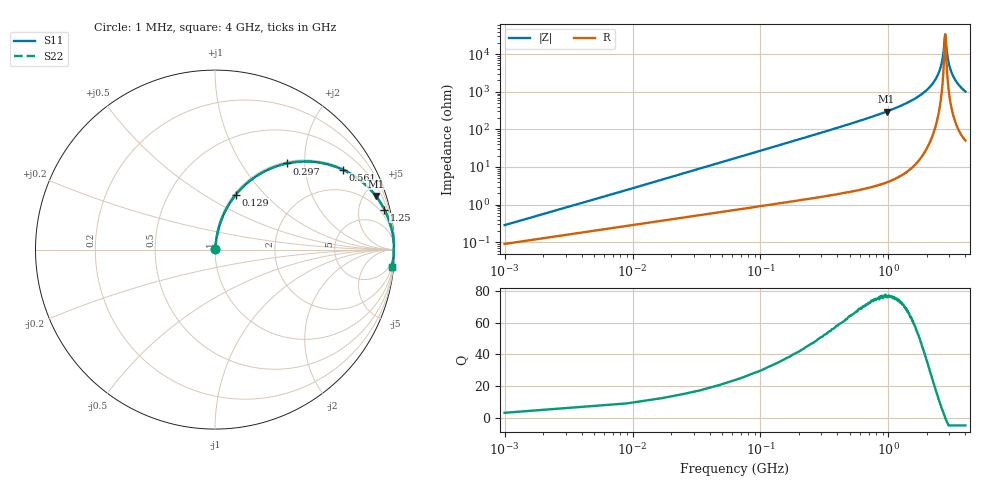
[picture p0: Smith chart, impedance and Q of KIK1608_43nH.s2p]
!version-2
!date-01.2022
!Series
# MHz S RI R 50
!Freq ReS11 ImS11 ReS21 ImS21 ReS12 ImS12 ReS22 ImS22
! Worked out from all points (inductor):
!   501 points, 1 MHz to 4 GHz, reference 50 ohm
!   read as one part in series: L = 43 nH near 17 MHz
!   highest Q = 76.7 at 969 MHz (marker M1), where L = 48.9 nH
!   self-resonance near 2.775 GHz
!   S11 on the Smith chart (normalised r, x): 1 MHz: 1.00, +0.01; 129 MHz: 1.02, +0.70; 297 MHz: 1.03, +1.62; 561 MHz: 1.05, +3.16; 1.25 GHz: 1.12, +8.45; 4 GHz: 2, -20
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1  0.000914 0.0027  0.9991 -0.0027  0.9991 -0.0027  0.000914 0.0027
25  0.009 0.0666  0.991 -0.0666  0.991 -0.0666  0.009 0.0666
41  0.0177 0.1082  0.9823 -0.1082  0.9823 -0.1082  0.0177 0.1082
73  0.0444 0.1872  0.9556 -0.1872  0.9556 -0.1872  0.0444 0.1872
129  0.1159 0.3056  0.8841 -0.3056  0.8841 -0.3056  0.1159 0.3056
297  0.3992 0.48  0.6008 -0.48  0.6008 -0.48  0.3992 0.48
561  0.7112 0.4458  0.2888 -0.4458  0.2888 -0.4458  0.7112 0.4458
673  0.7853 0.4037  0.2147 -0.4037  0.2147 -0.4037  0.7853 0.4037
969  0.8956 0.2993  0.1044 -0.2993  0.1044 -0.2993  0.8956 0.2993
1250  0.9442 0.2227  0.0558 -0.2227  0.0558 -0.2227  0.9442 0.2227
1335  0.954 0.2025  0.046 -0.2025  0.046 -0.2025  0.954 0.2025
2010  0.9898 0.0871  0.0102 -0.0871  0.0102 -0.0871  0.9898 0.0871
2450  0.9962 0.0339  0.00383 -0.0339  0.00383 -0.0339  0.9962 0.0339
2570  0.9968 0.0212  0.00322 -0.0212  0.00322 -0.0212  0.9968 0.0212
2670  0.997 0.0107  0.00298 -0.0107  0.00298 -0.0107  0.997 0.0107
2780  0.997 -0.00013  0.00298 0.00013  0.00298 0.00013  0.997 -0.00013
2810  0.997 -0.0024  0.00301 0.0024  0.00301 0.0024  0.997 -0.0024
2900  0.9968 -0.0113  0.00324 0.0113  0.00324 0.0113  0.9968 -0.0113
2980  0.9964 -0.0185  0.00356 0.0185  0.00356 0.0185  0.9964 -0.0185
3140  0.9955 -0.0323  0.00447 0.0323  0.00447 0.0323  0.9955 -0.0323
3335  0.994 -0.048  0.00603 0.048  0.00603 0.048  0.994 -0.048
4000  0.9856 -0.0966  0.0143 0.0966  0.0143 0.0966  0.9856 -0.0966
